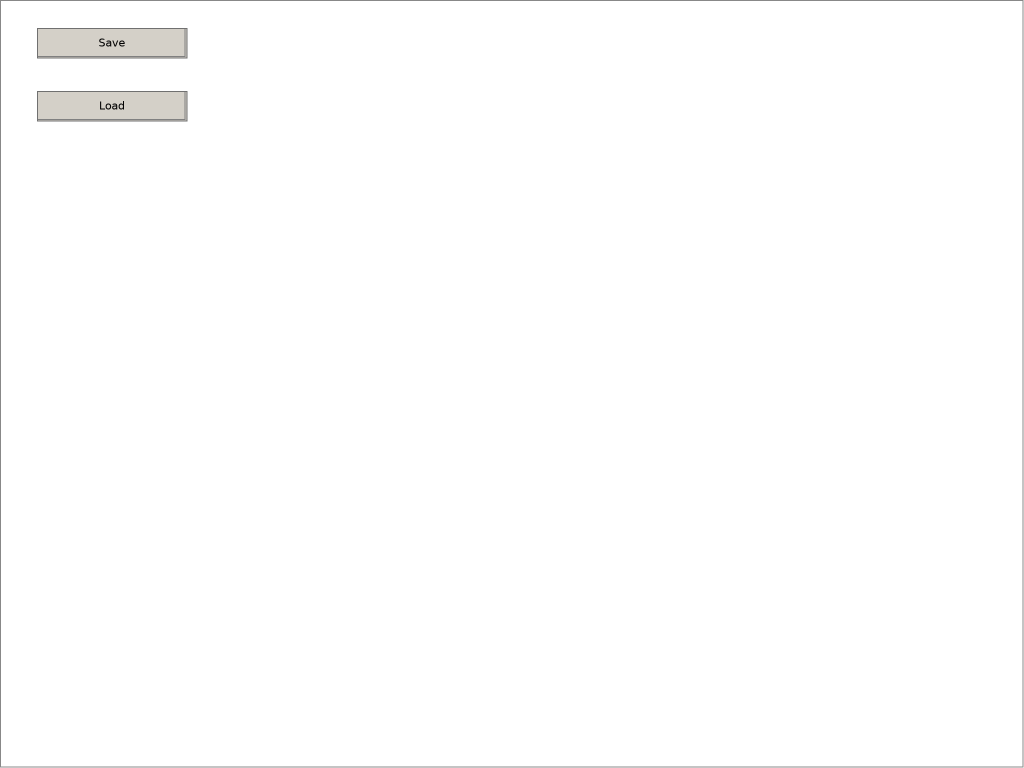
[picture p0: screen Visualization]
VISUALIZATION Visualization  // 1024x768
    Button (37,28 150x30), "Save"
        OnMouseClick: ExecuteCommand ExecuteCommand=ExecuteCommand=[Command=CreateRecipe, Value='Recipes', Value2='Test', Command=SaveRecipeAs, Value='Recipes', Value2='Test']
    Button (37,91 150x30), "Load"
        OnMouseClick: ExecuteCommand ExecuteCommand=ExecuteCommand=[Command=CreateRecipe, Value='Recipes', Value2='Test', Command=LoadRecipeFrom, Value='Recipes', Value2='Test']
END_VISUALIZATION
